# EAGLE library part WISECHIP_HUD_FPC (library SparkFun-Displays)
Kyocera 046288010000846+ - 10 Position Flat Flex Cable Connector for WiseChip HUD This 10 position FFC connects to the WiseChip transparent OLED HUD (Part Number: WiseChip US-0011 MIAG01, SFE SKU: LCD-14137) SparkFun Products: SparkX Qwiic Transparent OLED HUD
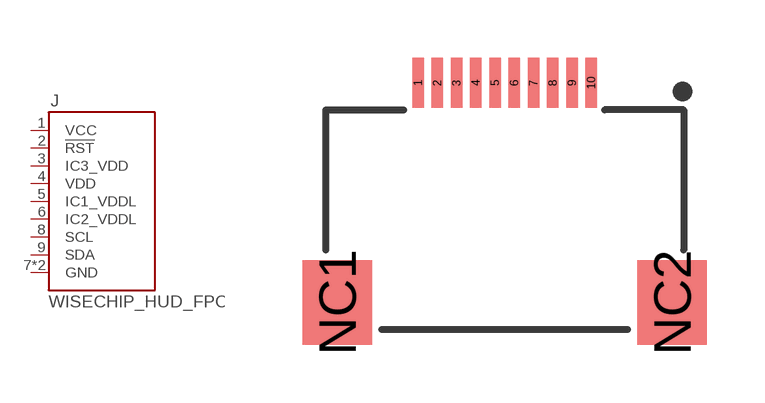
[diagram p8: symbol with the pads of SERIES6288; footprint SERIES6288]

Designator prefix J

## WISECHIP_HUD_FPC (PROD_ID: LCD-14137, CONN-14136)  [SERIES6288]
1  VCC
2  !RST
3  IC3_VDD
4  VDD
5  IC1_VDDL
6  IC2_VDDL
7  GND
8  SCL
9  SDA
10  GND

## Footprint SERIES6288 (pad centres in mm)
Kyocera 046288010000846+ - 10 Position Flat Flex Cable Connector for WiseChip HUD Specifications: Pin count: 10 Pin pitch: .5 mm Area: 10.5 mm x 7.45 mm Datasheet referenced for footprint
smd 0.3 x 1.3: 1 -2.3,3.4; 2 -1.8,3.4; 3 -1.3,3.4; 4 -0.8,3.4; 5 -0.3,3.4; 6 0.2,3.4; 7 0.7,3.4; 8 1.2,3.4; 9 1.7,3.4; 10 2.2,3.4
smd 1.8 x 2.2: NC1 -4.4,-2.3; NC2 4.3,-2.3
